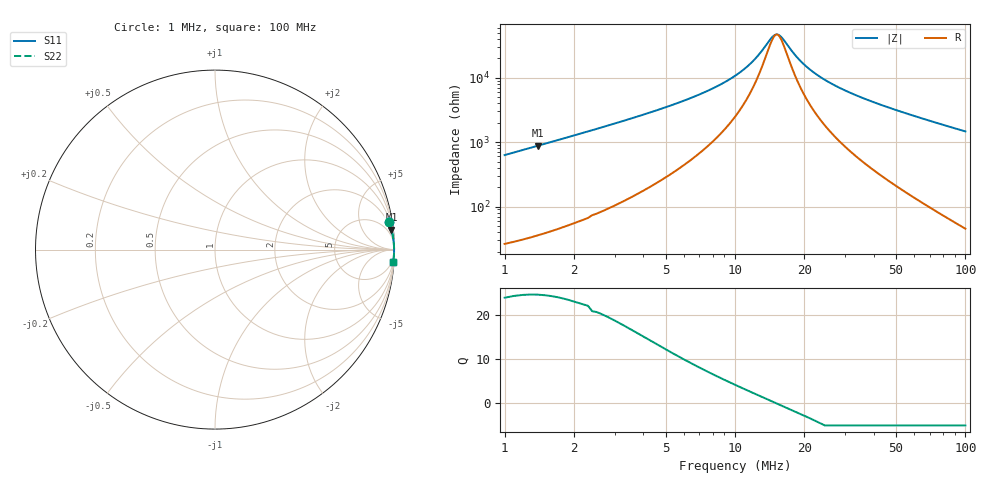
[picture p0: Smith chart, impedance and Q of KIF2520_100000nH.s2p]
!version-2
!date-12.2020
!Series
# MHz S RI R 50
!Freq ReS11 ImS11 ReS21 ImS21 ReS12 ImS12 ReS22 ImS22
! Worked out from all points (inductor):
!   991 points, 1 MHz to 100 MHz, reference 50 ohm
!   read as one part in series: L = 99.2 uH near 1.4 MHz
!   highest Q = 23.9 at 1.4 MHz (marker M1), where L = 100 uH
!   self-resonance near 15.1 MHz
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1  0.9693 0.153  0.0307 -0.153  0.0307 -0.153  0.9693 0.153
1.4  0.9829 0.1108  0.0171 -0.1108  0.0171 -0.1108  0.9829 0.1108
1.9  0.9897 0.0818  0.0103 -0.0818  0.0103 -0.0818  0.9897 0.0818
2.4  0.9927 0.0645  0.0073 -0.0645  0.0073 -0.0645  0.9927 0.0645
3.8  0.9959 0.0393  0.00405 -0.0393  0.00405 -0.0393  0.9959 0.0393
5.5  0.9971 0.0252  0.00293 -0.0252  0.00293 -0.0252  0.9971 0.0252
10.9  0.9978 0.00711  0.0022 -0.00711  0.0022 -0.00711  0.9978 0.00711
12.2  0.9978 0.00465  0.00216 -0.00465  0.00216 -0.00465  0.9978 0.00465
14.6  0.9979 0.000823  0.00213 -0.000823  0.00213 -0.000823  0.9979 0.000823
15.1  0.9979 0.000113  0.00212 -0.000113  0.00212 -0.000113  0.9979 0.000113
15.6  0.9979 -0.000574  0.00212 0.000574  0.00212 0.000574  0.9979 -0.000574
17.5  0.9979 -0.00301  0.00213 0.00301  0.00213 0.00301  0.9979 -0.00301
18.7  0.9979 -0.00443  0.00213 0.00443  0.00213 0.00443  0.9979 -0.00443
20  0.9979 -0.00589  0.00215 0.00589  0.00215 0.00589  0.9979 -0.00589
23.4  0.9978 -0.00941  0.0022 0.00941  0.0022 0.00941  0.9978 -0.00941
28  0.9977 -0.0137  0.00229 0.0137  0.00229 0.0137  0.9977 -0.0137
34  0.9975 -0.0189  0.00246 0.0189  0.00246 0.0189  0.9975 -0.0189
41.4  0.9973 -0.0249  0.00272 0.0249  0.00272 0.0249  0.9973 -0.0249
50.5  0.9969 -0.0319  0.00312 0.0319  0.00312 0.0319  0.9969 -0.0319
67  0.996 -0.0441  0.00405 0.0441  0.00405 0.0441  0.996 -0.0441
83.5  0.9948 -0.0559  0.00524 0.0559  0.00524 0.0559  0.9948 -0.0559
100  0.9933 -0.0675  0.00669 0.0675  0.00669 0.0675  0.9933 -0.0675
